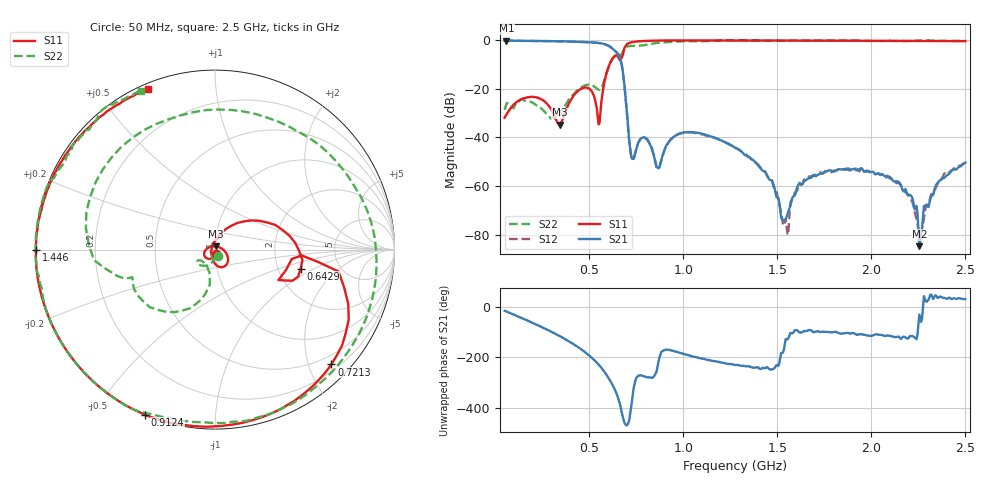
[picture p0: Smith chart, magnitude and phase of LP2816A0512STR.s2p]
!	AVX THIN FILM OPERATION
!	LP2816S High Performance Low Pass Filters
!	P/N LP2816S0512ANTR
! Created  22 November 2016
!Instrument: 	"HEWLETT PACKARD,8720ES,US39172150,7.62 "
# MHz S dB R 50
!  Frq	S11(dB)	S11(deg)	S21(dB)	S21(deg)	S12(dB)	S12(deg)	S22(dB)	S22(deg)
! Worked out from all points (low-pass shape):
!   501 points, 50 MHz to 2.5 GHz, reference 50 ohm
!   highest |S21| = -0.09 dB at 59.8 MHz (marker M1); lowest = -84.8 dB at 2.255 GHz (marker M2)
!   |S21| within 3 dB of the highest: start of sweep to 618.7 MHz
!   lowest |S11| = -34.7 dB at 344 MHz (marker M3), VSWR 1.04, Z = 50.3 + j1.81 ohm
!   |S11| at or under -10 dB: start of sweep to 607.3 MHz
!   |S22| runs from -32.4 to 0.0 dB; largest |S21 - S12| = 0.017
!   S11 on the Smith chart (normalised r, x): 50 MHz: 1.01, -0.05; 642.9 MHz: 2.67, -0.74; 721.3 MHz: 0.32, -2.40; 912.4 MHz: 0.00, -0.66; 1.446 GHz: 0.00, -0.00; 2.5 GHz: 0.02, +0.67
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50  -31.85 -82.4  -0.11 -16.1  -0.10 -15.9  -28.62 -67.3
59.8  -30.52 -88.4  -0.09 -19.0  -0.09 -19.2  -26.10 -76.3
211.7  -23.36 -150.6  -0.23 -68.3  -0.20 -68.3  -26.28 -112.1
344  -34.72 79.0  -0.35 -116.9  -0.34 -117.0  -30.57 -107.7
461.6  -19.72 -49.7  -0.59 -171.1  -0.61 -171.6  -19.14 -125.5
549.8  -34.56 178.2  -1.03 130.7  -1.05 130.2  -20.40 -135.7
642.9  -6.22 -12.5  -4.75 19.4  -4.68 17.9  -6.15 -144.2
677.2  -6.30 -3.8  -12.03 -72.8  -12.24 -75.0  -5.00 -164.8
721.3  -0.81 -44.6  -47.00 -46.8  -46.84 -42.7  -2.25 138.5
780.1  -0.26 -75.5  -40.18 86.8  -40.34 86.7  -2.06 73.2
868.3  -0.05 -102.8  -52.72 142.8  -53.00 145.3  -0.95 0.1
912.4  0.00 -112.9  -43.01 -170.3  -43.12 -167.2  -0.67 -25.8
1044.7  0.00 -136.2  -37.77 163.6  -37.90 166.3  -0.27 -80.7
1275  0.00 -164.1  -44.27 128.5  -44.14 130.6  0.00 -132.7
1446.5  -0.02 -179.9  -55.92 120.8  -55.74 118.1  0.00 -156.4
1549.4  -0.03 171.8  -72.68 -128.8  -76.82 -126.9  -0.06 -169.4
1686.6  -0.07 161.7  -55.95 -97.9  -55.94 -91.6  0.00 177.1
2093.3  -0.19 135.5  -56.52 -114.4  -56.09 -113.6  -0.14 143.1
2210.9  -0.20 128.7  -64.05 -116.2  -65.61 -114.6  -0.21 133.6
2255  -0.22 126.2  -84.80 -30.9  -80.38 -53.4  -0.08 130.3
2362.8  -0.25 120.2  -57.84 40.2  -57.94 41.4  -0.09 124.5
2500  -0.28 112.7  -50.36 30.6  -50.46 30.9  -0.21 114.8
